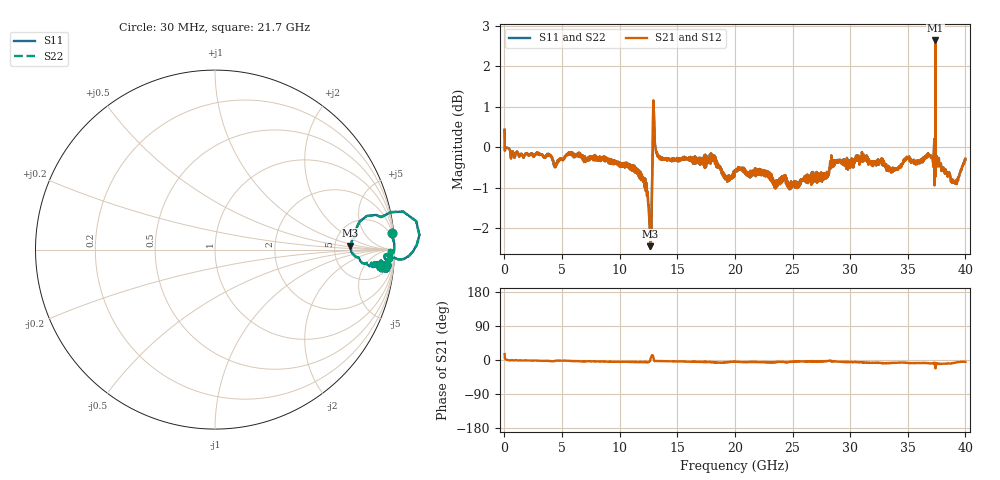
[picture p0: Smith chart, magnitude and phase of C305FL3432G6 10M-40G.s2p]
!Agilent Technologies,N5234A,MY52241123,A.10.00.00
!Agilent N5234A: A.10.00.00
!Date: Wednesday, February 02, 2022 09:21:19
!Correction: S11(Response(S21))
!S21(Response(S21))
!S12(Response(S21))
!S22(Response(S21))
!S2P File: Measurements: S11, S21, S12, S22:
# Hz S  dB  R 50
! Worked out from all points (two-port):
!   2001 points, 10 MHz to 40 GHz, reference 50 ohm
!   highest |S21| = 2.64 dB at 37.4 GHz (marker M1); lowest = -2.4 dB at 12.67 GHz (marker M2)
!   |S21| within 3 dB of the highest: start of sweep to 4.242 GHz; 4.584 GHz to 9.01 GHz (4.426 GHz wide, 65.1 % of centre)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
!   lowest |S11| = -2.4 dB at 12.67 GHz (marker M3), VSWR 7.16, Z = 354 + j37.5 ohm
!   |S11| at or under -10 dB: nowhere
!   |S22| runs from -2.4 to 2.6 dB; largest |S21 - S12| = 0
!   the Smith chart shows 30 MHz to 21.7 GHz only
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1e7  0.43 15.5  0.43 15.5  0.43 15.5  0.43 15.5
2.29945e8  -0.01 0.2  -0.01 0.2  -0.01 0.2  -0.01 0.2
3.89905e8  -0.03 -0.6  -0.03 -0.6  -0.03 -0.6  -0.03 -0.6
6.68833e9  -0.24 -3.8  -0.24 -3.8  -0.24 -3.8  -0.24 -3.8
1.070732e10  -0.41 -5.0  -0.41 -5.0  -0.41 -5.0  -0.41 -5.0
1.232692e10  -0.89 -6.0  -0.89 -6.0  -0.89 -6.0  -0.89 -6.0
1.250688e10  -1.42 -5.0  -1.42 -5.0  -1.42 -5.0  -1.42 -5.0
1.266684e10  -2.44 1.7  -2.44 1.7  -2.44 1.7  -2.44 1.7
1.28268e10  -0.52 11.1  -0.52 11.1  -0.52 11.1  -0.52 11.1
1.300675e10  0.45 -2.8  0.45 -2.8  0.45 -2.8  0.45 -2.8
1.314672e10  -0.08 -2.9  -0.08 -2.9  -0.08 -2.9  -0.08 -2.9
1.334666e10  -0.21 -2.9  -0.21 -2.9  -0.21 -2.9  -0.21 -2.9
1.864534e10  -0.50 -7.0  -0.50 -7.0  -0.50 -7.0  -0.50 -7.0
2.0005e10  -0.59 -4.5  -0.59 -4.5  -0.59 -4.5  -0.59 -4.5
2.310422e10  -0.70 -6.9  -0.70 -6.9  -0.70 -6.9  -0.70 -6.9
2.668333e10  -0.61 -3.7  -0.61 -3.7  -0.61 -3.7  -0.61 -3.7
2.814296e10  -0.68 -2.1  -0.68 -2.1  -0.68 -2.1  -0.68 -2.1
3.112222e10  -0.17 -6.4  -0.17 -6.4  -0.17 -6.4  -0.17 -6.4
3.334166e10  -0.49 -8.5  -0.49 -8.5  -0.49 -8.5  -0.49 -8.5
3.740065e10  2.64 -22.1  2.64 -22.1  2.64 -22.1  2.64 -22.1
3.894026e10  -0.87 -7.9  -0.87 -7.9  -0.87 -7.9  -0.87 -7.9
4e10  -0.29 -4.8  -0.29 -4.8  -0.29 -4.8  -0.29 -4.8
